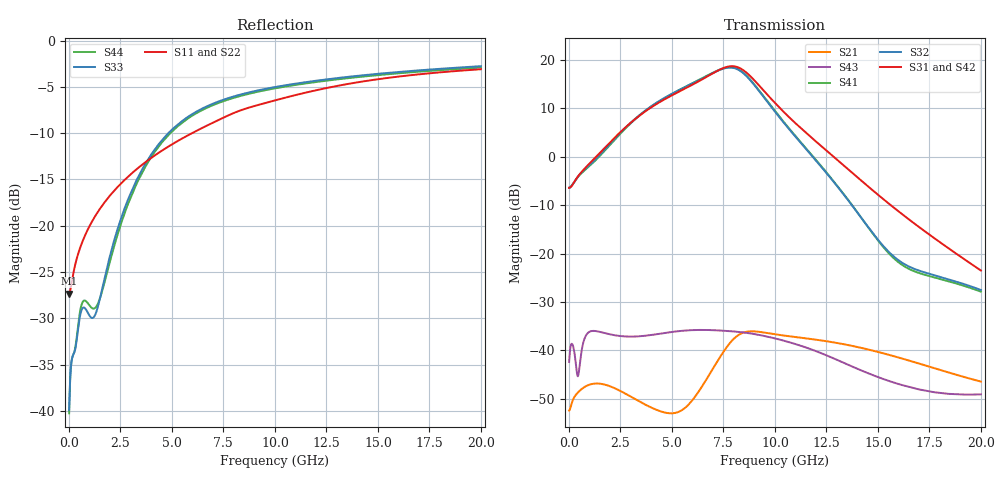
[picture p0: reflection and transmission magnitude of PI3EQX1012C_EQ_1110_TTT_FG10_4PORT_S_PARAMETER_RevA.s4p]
! NPort=4 DATA=2000 NOISE=0 GROUPDELAY=0 COMPLEX_DATAFORMAT=POLAR
! NumOfBlock=1 NumOfParam=0
! .MODEL Smodel S TSTONEFILE=PI3EQX1012C_EQ_1110_TTT_FG10_4PORT_S_PARAMETER_RevA.s4p TYPE=S
!  -- The above .MODEL line can be used for the S element in the netlist.
! The s parameter is extracted from the linear redriver, it is not bi-directional; only s(4,1)s(4,2) and s(3,1)s(3,2)
! should be the insertion loss
!Port definition:
!Port1 = input+
!Port2 = input-
!Port3 = output+
!Port4 = output-
# Hz S MA R  50
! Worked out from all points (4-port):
!   2000 points, 10 MHz to 20 GHz, reference 50 ohm
!   strongest paths, dB at 10 MHz, 5.01 GHz, 10.01 GHz, 15.01 GHz, 20 GHz:
!     S31: -6.4, 12.7, 11.1, -7.9, -23.5
!     S42: -6.4, 12.7, 11.1, -7.7, -23.1
!     S32: -6.4, 13.0, 9.3, -17.2, -27.5
!     S41: -6.4, 13.0, 9.4, -17.3, -27.9
!     S43: -42.4, -36.2, -37.5, -45.5, -49.1
!     S21: -52.4, -53.0, -36.7, -40.3, -46.4
!   lowest |S11| = -27.3 dB at 10 MHz (marker M1), VSWR 1.09, Z = 45.9 - j0.123 ohm
!   |S11| at or under -10 dB: start of sweep to 5.978 GHz
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1e7  0.04301 -178.2  0.002379 1.5  0.0008102 -0.5  0.0008039 -0.5
     0.002388 1.5  0.04109 -178.1  0.000927 -0.5  0.0009197 -0.5
     0.4788 0.4  0.4779 -179.5  0.01016 -4.0  0.007598 -25.7
     0.4774 -179.5  0.4797 0.4  0.007614 -25.8  0.009722 -4.0
5.77e9  0.3074 -123.6  0.002827 56.8  0.0002773 -58.3  0.0002761 -59.2
        0.002702 54.5  0.3124 -122.9  0.0003144 -59.2  0.0003132 -60.2
        5.239 -129.9  5.413 58.2  0.3866 -99.6  0.01646 9.2
        5.433 58.5  5.257 -128.0  0.01609 6.6  0.3789 -99.4
7.24e9  0.3713 -124.2  0.008322 70.1  0.0002366 -55.5  0.0002344 -56.9
        0.007903 71.3  0.3766 -123.8  0.0002667 -56.8  0.0002643 -58.1
        7.781 158.9  7.756 -14.2  0.4677 -110.8  0.01669 -13.7
        7.824 -14.4  7.818 161.0  0.01608 -14.0  0.4593 -110.6
8.15e9  0.4125 -125.8  0.01444 44.7  0.0002247 -54.2  0.0002217 -55.7
        0.014 46.5  0.4183 -125.3  0.0002518 -55.6  0.0002484 -57.1
        8.477 97.0  8.062 -77.0  0.5046 -116.1  0.01586 -26.1
        8.154 -77.4  8.518 99.3  0.01558 -25.7  0.4959 -116.0
9.04e9  0.4441 -127.8  0.01596 14.6  0.0002177 -53.8  0.0002139 -55.4
        0.01569 16.2  0.4509 -127.3  0.0002425 -55.1  0.0002384 -56.6
        6.041 37.7  5.378 -136.8  0.5339 -120.4  0.01485 -36.7
        5.452 -137.5  6.07 40.2  0.01469 -37.1  0.5252 -120.2
1.065e10  0.4963 -130.2  0.01411 -14.0  0.0002091 -55.0  0.0002045 -56.5
          0.01403 -12.9  0.5041 -129.8  0.0002316 -55.9  0.0002267 -57.5
          2.61 -32.6  1.974 153.9  0.5769 -126.3  0.01249 -54.5
          2.007 152.4  2.625 -29.6  0.01222 -55.2  0.5679 -126.2
2e10  0.7001 -144.7  0.004849 -76.3  0.0001462 -72.3  0.0001411 -73.8
      0.004763 -75.3  0.7152 -144.4  0.0001621 -72.1  0.0001564 -73.8
      0.06681 99.9  0.04206 27.7  0.7272 -143.5  0.003595 -51.4
      0.04045 26.3  0.06998 104.8  0.003514 -48.7  0.7152 -143.3
